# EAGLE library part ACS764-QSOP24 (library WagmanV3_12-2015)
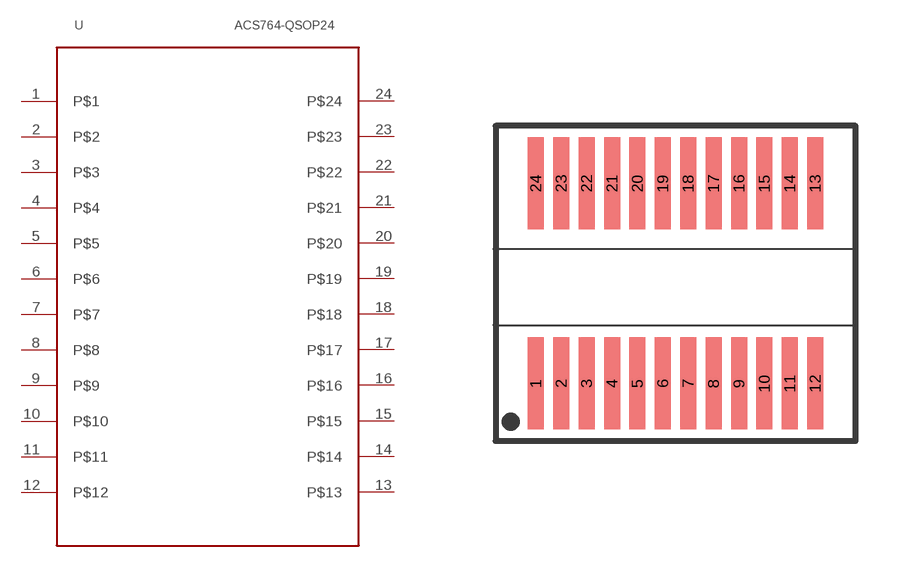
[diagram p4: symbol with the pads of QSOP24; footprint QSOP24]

Designator prefix U

## ACS764-QSOP24  [QSOP24]
1  P$1
2  P$2
3  P$3
4  P$4
5  P$5
6  P$6
7  P$7
8  P$8
9  P$9
10  P$10
11  P$11
12  P$12
13  P$13
14  P$14
15  P$15
16  P$16
17  P$17
18  P$18
19  P$19
20  P$20
21  P$21
22  P$22
23  P$23
24  P$24

## Footprint QSOP24 (pad centres in mm)
24-Lead Quarter Size Outline Q13 Source: www.cypress.com .. CY7C6301XX.pdf
smd 0.4 x 2.3: 1 -3.493,-2.5; 2 -2.857,-2.5; 3 -2.223,-2.5; 4 -1.587,-2.5; 5 -0.953,-2.5; 6 -0.318,-2.5; 7 0.318,-2.5; 8 0.953,-2.5; 9 1.587,-2.5; 10 2.223,-2.5; 11 2.857,-2.5; 12 3.493,-2.5; 13 3.493,2.5; 14 2.857,2.5; 15 2.223,2.5; 16 1.587,2.5; 17 0.953,2.5; 18 0.318,2.5; 19 -0.318,2.5; 20 -0.953,2.5; 21 -1.587,2.5; 22 -2.223,2.5; 23 -2.857,2.5; 24 -3.493,2.5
